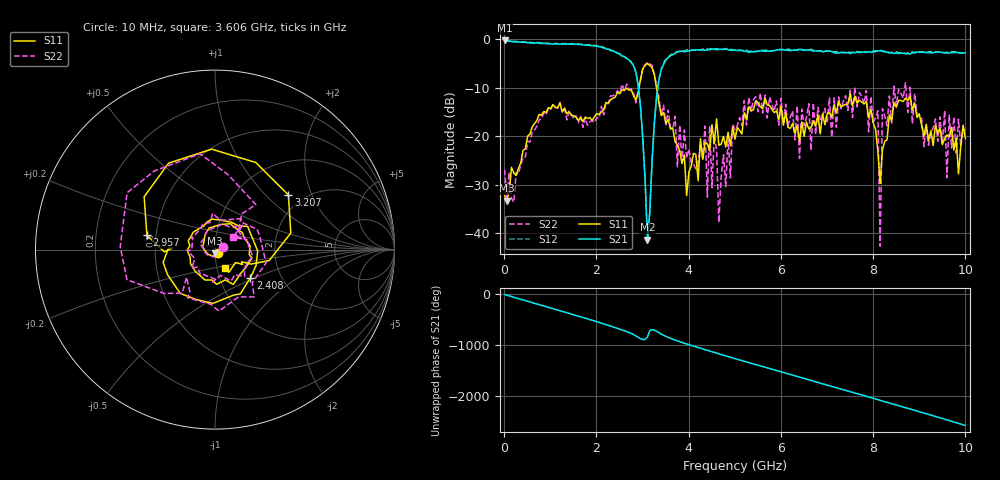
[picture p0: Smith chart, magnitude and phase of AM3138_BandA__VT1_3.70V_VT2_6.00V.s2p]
! Date/Time: Tue, Nov 13, 2018 4:43 PM
! Network Analyzer: Agilent Technologies E8364B Rev: A.07.50.67
! Sweep from 0.010 to 10.000 GHz, 201 Points, Sweep Type: LIN
! Power Supply: 3.701 V, 0.000 A
# Hz S DB R 50
!freq MagS11 AngS11 MagS21 AngS21 MagS12 AngS12 MagS22 AngS22
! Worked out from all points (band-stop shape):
!   201 points, 10 MHz to 10 GHz, reference 50 ohm
!   highest |S21| = -0.26 dB at 10 MHz (marker M1); lowest = -41.4 dB at 3.107 GHz (marker M2)
!   |S21| within 3 dB of the highest: start of sweep to 2.529 GHz; 3.641 GHz to end of sweep
!   lowest |S11| = -33.3 dB at 59.95 MHz (marker M3), VSWR 1.04, Z = 49.9 - j2.15 ohm
!   |S11| at or under -10 dB: start of sweep to 2.925 GHz; 3.303 GHz to end of sweep
!   |S22| runs from -42.7 to -4.7 dB; largest |S21 - S12| = 0.027
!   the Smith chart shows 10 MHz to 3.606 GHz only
!   S11 on the Smith chart (normalised r, x): 10 MHz: 1.04, -0.03; 2.408 GHz: 1.40, -0.47; 2.957 GHz: 0.44, +0.08; 3.207 GHz: 1.67, +1.38; 3.606 GHz: 1.10, -0.23
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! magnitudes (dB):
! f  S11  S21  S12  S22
! 10 MHz  -32.2  -0.3  -0.3  -26.9
! 59.95 MHz  -33.3  -0.4  -0.3  -32.9
! 1.708 GHz  -17.0  -1.1  -1.1  -18.2
! 2.408 GHz  -12.0  -2.7  -2.6  -11.3
! 2.957 GHz  -8.2  -14.0  -14.0  -8.5
! 3.107 GHz  -5.0  -41.4  -42.0  -4.7
! 3.207 GHz  -5.9  -25.2  -25.1  -5.3
! 3.357 GHz  -13.3  -8.3  -8.3  -12.1
! 3.606 GHz  -18.5  -3.4  -3.3  -18.2
! 3.956 GHz  -32.3  -2.5  -2.2  -24.5
! 4.356 GHz  -21.3  -2.3  -2.0  -17.9
! 4.406 GHz  -21.5  -2.2  -2.0  -32.6
! 4.456 GHz  -23.1  -2.2  -2.1  -17.9
! 4.655 GHz  -21.9  -2.1  -2.1  -37.8
! 5.005 GHz  -20.6  -2.3  -2.2  -18.7
! 6.703 GHz  -16.9  -2.5  -2.2  -13.1
! 8.102 GHz  -23.1  -2.4  -2.3  -14.7
! 8.152 GHz  -29.7  -2.4  -2.3  -42.7
! 8.202 GHz  -22.8  -2.5  -2.4  -14.3
! 8.352 GHz  -15.6  -2.8  -2.8  -11.7
! 9.6 GHz  -19.8  -2.8  -2.7  -28.6
! 10 GHz  -20.5  -2.8  -2.7  -18.8
